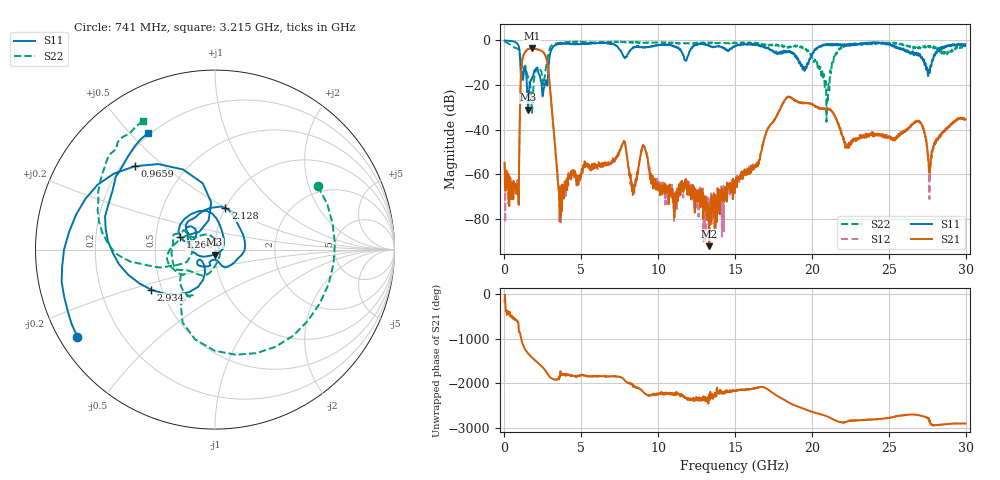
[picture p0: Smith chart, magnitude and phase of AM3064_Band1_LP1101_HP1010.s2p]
# Hz S DB R 50.0
!freq dBS11 angS11 dBS21 angS21 dBS12 angS12 dBS22 angS22
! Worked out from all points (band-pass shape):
!   1600 points, 10 MHz to 29.98 GHz, reference 50 ohm
!   highest |S21| = -3.49 dB at 1.791 GHz (marker M1); lowest = -92.3 dB at 13.3 GHz (marker M2)
!   |S21| within 3 dB of the highest: 1.242 GHz to 2.641 GHz (1.399 GHz wide, 72 % of centre)
!   lowest |S11| = -31.1 dB at 1.547 GHz (marker M3), VSWR 1.06, Z = 49.7 - j2.76 ohm
!   |S11| at or under -10 dB: 1.031 GHz to 2.893 GHz (1.862 GHz wide, 94.9 % of centre); 19.24 GHz to 19.79 GHz (549.8 MHz wide, 2.82 % of centre); 27.3 GHz to 27.79 GHz (489.7 MHz wide, 1.78 % of centre)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
!   |S22| runs from -36.5 to -0.4 dB; largest |S21 - S12| = 0.0083
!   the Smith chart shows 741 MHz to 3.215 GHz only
!   S11 on the Smith chart (normalised r, x): 741 MHz: 0.05, -0.29; 965.9 MHz: 0.25, +0.40; 1.266 GHz: 0.67, +0.10; 2.128 GHz: 1.00, +0.49; 2.934 GHz: 0.44, -0.24; 3.215 GHz: 0.19, +0.56
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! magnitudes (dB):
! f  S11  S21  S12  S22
! 10 MHz  0.0  -54.8  -54.8  -0.4
! 741 MHz  -0.8  -65.0  -67.3  -3.4
! 965.9 MHz  -3.8  -48.7  -48.8  -5.0
! 1.266 GHz  -13.7  -6.1  -6.1  -12.4
! 1.547 GHz  -31.1  -3.9  -3.8  -17.1
! 1.791 GHz  -16.9  -3.5  -3.5  -32.5
! 2.128 GHz  -12.5  -4.0  -4.0  -12.2
! 2.934 GHz  -7.5  -18.8  -18.7  -3.9
! 3.215 GHz  -2.5  -41.8  -41.4  -1.7
! 3.646 GHz  -1.5  -78.6  -65.3  -1.0
! 5.015 GHz  -1.6  -59.2  -59.5  -0.5
! 7.732 GHz  -6.9  -45.6  -45.7  -0.7
! 10 GHz  -2.1  -63.8  -67.0  -0.9
! 13.3 GHz  -2.4  -92.3  -74.5  -1.2
! 15 GHz  -2.7  -63.4  -65.4  -1.3
! 19.99 GHz  -6.9  -28.7  -28.6  -6.8
! 20.98 GHz  -1.7  -30.9  -30.6  -26.1
! 21.9 GHz  -2.1  -40.7  -41.9  -2.8
! 25 GHz  -1.4  -43.5  -42.8  -1.3
! 26.98 GHz  -6.9  -36.5  -36.4  -2.9
! 27.68 GHz  -13.6  -56.5  -61.3  -2.6
! 29.98 GHz  -1.6  -35.4  -35.3  -2.9
